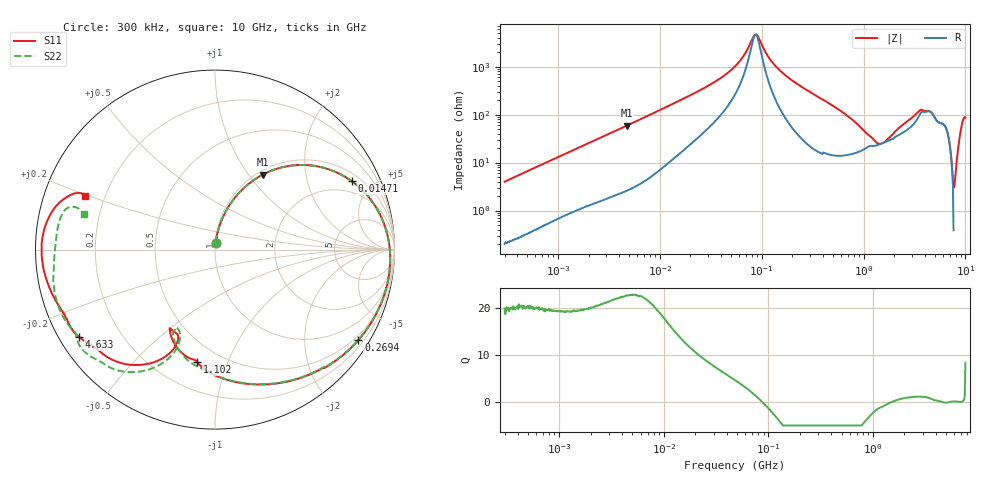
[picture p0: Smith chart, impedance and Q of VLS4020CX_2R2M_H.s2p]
! S-Parameter Data Generated by TDK Corporation
! Copyright(C) 2024 TDK Corporation.
! All Rights Reserved.
! TDK P/N: VLS4020CX-2R2M-H (SMD / SMT Inductor (Coil))
! Property: L=2.2uH at 1MHz
! Size(LxWxT): 4x4x2mm
! Model Type: s2p (Touchstone File Format Version 1.0)
! Frequency: DC=Yes Start=0.3MHz Stop=10000MHz 802points Log-sweep
! Model Generated on May 28, 2024
! Terms and conditions regarding TDK Simulation Models:
! 1)This simulation model is being provided solely for informational
!  purposes. Please refer to the specifications of the products in
!  terms of detailed characteristics of such products.
! 2)In no event shall TDK Corporation of any of its subsidiaries be
!  liable for any loss or damage arising, directly or indirectly,
!  from any information contained in this simulation model, including,
!  but not limited to loss or damages arising from any inaccuracies,
!  omissions or errors in connection with such information.
! 3)Any and all copyrights on this simulation model are owned by
!  TDK Corporation.  Duplication or redistribution of this simulation
!  model without prior written permission from TDK Corporation
!  is prohibited.
! 4)This simulation model is subject to any modification or change
!  without any prior notice.
! 5)Neither TDK Corporation nor any of its subsidiaries shall make any
!  warranty, express or implied, including but not limited to the
!  correctness, implied warranties of merchantability and fitness for
!  a particular purpose with respect to this simulation models.
! 6)The use of this simulation model shall be deemed to have consented
!  to the terms and conditions hereof.
! Port Assignments:
!  1 ---@@@--- 2
! Applicable Conditions:
!  Temperature = 25 degC
!  DC Bias Current = 0 A
!  Small Signal Operation
# Hz S MA R 50
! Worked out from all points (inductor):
!   801 points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, 300 kHz to 10 GHz, reference 50 ohm
!   read as one part in series: L = 2.11 uH near 318.3 kHz
!   highest Q = 22.7 at 4.735 MHz (marker M1), where L = 1.97 uH
!   self-resonance near 87.3 MHz
!   S11 on the Smith chart (normalised r, x): 300 kHz: 1.00, +0.08; 14.71 MHz: 1.36, +3.77; 269.4 MHz: 0.37, -3.42; 1.102 GHz: 0.37, -0.78; 4.633 GHz: 0.06, -0.29; 10 GHz: 0.13, +0.20
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300000  0.03947 84.8  0.9973 -2.3  0.9971 -2.3  0.03941 84.8
1713600  0.2097 74.9  0.9672 -12.2  0.967 -12.2  0.2096 74.9
4734969  0.4953 57.5  0.8473 -29.9  0.847 -29.9  0.4953 57.5
9671944  0.7473 38.0  0.6248 -48.9  0.6247 -48.9  0.7472 38.0
1.470778e7  0.8517 26.6  0.4642 -59.1  0.4641 -59.1  0.8517 26.6
5.477226e7  0.9709 1.8  0.09582 -73.2  0.09582 -73.2  0.9709 1.9
8.857507e7  0.9792 -5.8  0.02089 2.1  0.0209 2.1  0.9792 -5.7
1.454054e8  0.9758 -15.3  0.1068 65.0  0.1068 64.9  0.9757 -15.1
2.694285e8  0.9445 -32.3  0.262 53.7  0.2619 53.7  0.9445 -31.9
3.126428e8  0.9299 -37.6  0.3057 48.7  0.3056 48.7  0.9301 -37.2
5.82867e8  0.8221 -65.1  0.4906 20.3  0.4906 20.3  0.8231 -64.3
1.10164e9  0.6357 -98.9  0.5952 -23.0  0.5949 -23.0  0.6613 -97.7
1.767019e9  0.5246 -118.5  0.5716 -66.2  0.572 -66.2  0.5214 -116.7
2.172958e9  0.5219 -113.3  0.5 -91.9  0.5007 -91.9  0.4908 -114.2
2.69003e9  0.6426 -114.2  0.3542 -122.5  0.3549 -122.6  0.6263 -112.0
3.387826e9  0.8189 -129.3  0.1607 -147.5  0.1608 -147.7  0.8327 -124.9
4.632637e9  0.9002 -147.2  0.07517 -125.7  0.07487 -125.5  0.9254 -143.6
5.445625e9  0.913 -154.1  0.08253 -127.9  0.08235 -127.9  0.9046 -149.1
6.253087e9  0.926 -160.6  0.06006 -139.4  0.05996 -139.3  0.9237 -155.3
7.652089e9  0.9662 180.0  0.04304 -130.3  0.04304 -130.2  0.8996 -175.7
9.105558e9  0.8866 161.4  0.03905 -129.9  0.03897 -129.7  0.8696 165.9
1e10  0.782 157.5  0.0388 -121.5  0.03879 -121.4  0.7537 165.0
